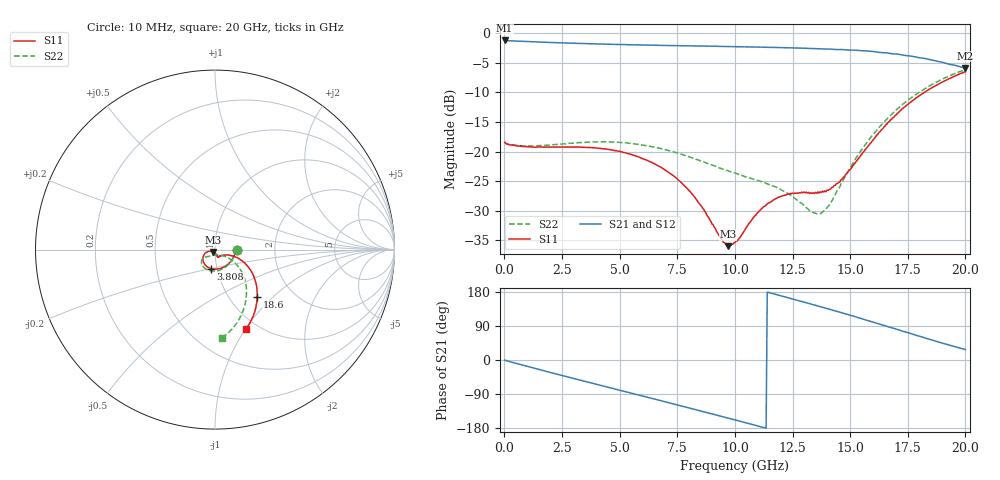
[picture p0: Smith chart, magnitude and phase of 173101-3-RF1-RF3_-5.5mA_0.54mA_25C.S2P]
!  2-Port S-parameters saved by WinCal
! VAR MeasName=S-Parameters (CALIBRATED_DATA) read from VNA (N5242A)
! VAR MeasDate=2017-7-20 9:26:34
! VAR NAME=173101-3-RF1-RF3_-5.5mA_0.54mA_25C
! VAR FILENAME=173101-3-RF1-RF3_-5.5mA_0.54mA_25C.S2P
! VAR DATE=2017-7-20 9:26:34
! VAR PHYS_PORTS=1,2
# Hz S DB R 50
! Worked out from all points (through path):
!   401 points, 10 MHz to 20 GHz, reference 50 ohm
!   highest |S21| = -1.20 dB at 10 MHz (marker M1); lowest = -5.9 dB at 20 GHz (marker M2)
!   group delay of S21, straight-line fit = 45.7 ps
!   lowest |S11| = -36.0 dB at 9.705 GHz (marker M3), VSWR 1.03, Z = 49.1 - j1.32 ohm
!   |S11| at or under -10 dB: start of sweep to 18.21 GHz
!   |S22| runs from -30.5 to -6.1 dB; largest |S21 - S12| = 0.0077
!   S11 on the Smith chart (normalised r, x): 10 MHz: 1.27, -0.00; 3.808 GHz: 0.94, -0.20; 18.6 GHz: 1.34, -0.80; 20 GHz: 0.89, -1.00
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1e7  -18.43 -0.8  -1.20 -0.3  -1.19 -0.3  -18.38 -0.7
1.559225e9  -19.21 -49.5  -1.47 -26.0  -1.47 -26.0  -18.98 -48.4
3.358325e9  -19.26 -92.8  -1.72 -54.3  -1.72 -54.3  -18.46 -88.2
3.8081e9  -19.33 -102.1  -1.76 -61.3  -1.76 -61.2  -18.36 -96.3
5.257375e9  -20.22 -128.6  -1.91 -83.7  -1.92 -83.6  -18.53 -118.0
6.70665e9  -22.46 -150.5  -2.02 -106.2  -2.01 -106.0  -19.39 -134.0
8.10595e9  -27.00 -163.3  -2.12 -128.0  -2.13 -127.8  -21.00 -143.0
9.4053e9  -34.83 -141.4  -2.21 -148.5  -2.20 -148.4  -22.85 -143.8
9.70515e9  -36.00 -122.1  -2.22 -153.3  -2.22 -153.2  -23.25 -143.2
1.0005e10  -35.36 -101.2  -2.25 -158.1  -2.25 -158.0  -23.62 -141.9
1.095452e10  -30.46 -72.6  -2.31 -173.4  -2.32 -173.2  -24.86 -137.1
1.155422e10  -28.50 -70.6  -2.36 176.8  -2.37 177.0  -25.70 -133.6
1.24038e10  -27.09 -70.9  -2.45 162.7  -2.44 162.9  -27.32 -125.3
1.335332e10  -27.09 -62.6  -2.56 146.8  -2.54 146.9  -30.21 -99.2
1.370315e10  -26.80 -54.9  -2.61 140.7  -2.63 140.8  -30.51 -79.9
1.405298e10  -26.55 -46.9  -2.66 134.9  -2.68 135.0  -29.23 -59.6
1.465268e10  -24.64 -31.3  -2.73 124.3  -2.75 124.6  -25.19 -38.0
1.54023e10  -20.96 -20.9  -2.90 110.9  -2.90 110.9  -20.24 -32.2
1.670165e10  -14.89 -24.2  -3.36 86.8  -3.40 86.9  -14.09 -40.3
1.76012e10  -11.70 -34.3  -3.83 70.4  -3.82 70.6  -11.03 -51.3
1.86007e10  -9.07 -48.0  -4.57 51.7  -4.60 52.0  -8.55 -65.2
2e10  -6.51 -68.5  -5.86 27.5  -5.90 28.1  -6.14 -85.5
